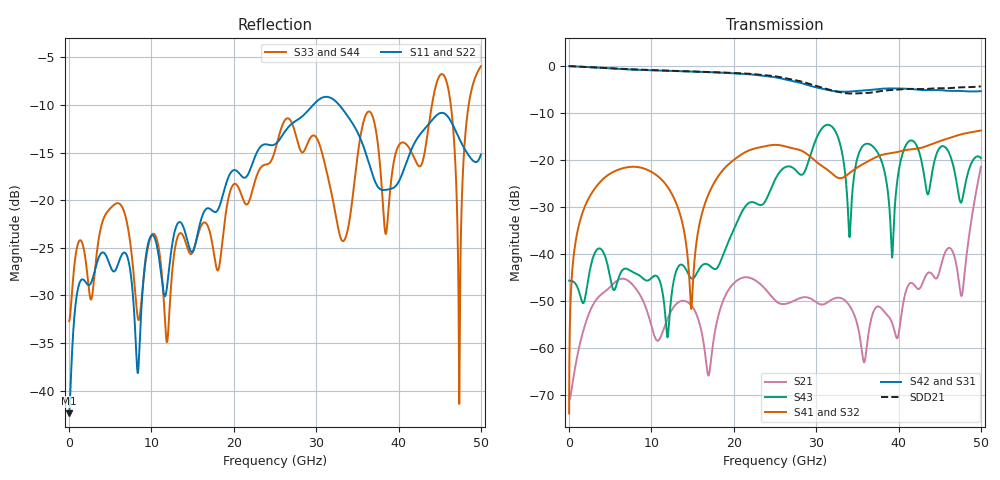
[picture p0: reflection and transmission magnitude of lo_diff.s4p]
!Keysight Technologies,N5245B,MY57181346,A.12.70.07
!Automatic Fixture Removal (AFR)
!Date: Tuesday, November 06, 2018 3:00:35 PM
!S4P File: Measurements: <S11,S12,S13,S14>,
!<S21,S22,S23,S24>,
!<S31,S32,S33,S34>,
!<S41,S42,S43,S44>:
# MHz S  RI  R 50
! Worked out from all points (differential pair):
!   5000 points, 10 MHz to 50 GHz, reference 50 ohm
!   strongest paths, dB at 10 MHz, 12.51 GHz, 25.01 GHz, 37.51 GHz, 50 GHz:
!     S42: 0.0, -1.0, -2.4, -4.9, -5.3
!     S31: 0.0, -1.0, -2.4, -4.9, -5.3
!     S41: -73.9, -27.3, -16.8, -19.2, -13.7
!     S32: -73.9, -27.3, -16.8, -19.2, -13.7
!     S43: -45.7, -47.9, -24.2, -18.5, -19.6
!     S21: -71.0, -51.8, -49.9, -51.2, -21.4
!   taken as a pair (ports 2,1 in; 4,3 out), SDD21 dB: 0.0, -1.0, -2.2, -5.4, -4.3
!   lowest |S11| = -42.4 dB at 10 MHz (marker M1), VSWR 1.02, Z = 50.8 + j0.0342 ohm
!   |S11| at or under -10 dB: start of sweep to 29.63 GHz; 32.8 GHz to end of sweep
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10  0.00759 0.000337  0.000282 4.52e-06  0.9997 -0.00825  0.000108 0.000169
    0.000282 4.52e-06  0.00759 0.000337  0.000108 0.000169  0.9997 -0.00825
    0.9997 -0.00825  0.000108 0.000169  0.0232 0.0004  -0.0052 9.39e-05
    0.000108 0.000169  0.9997 -0.00825  -0.0052 9.39e-05  0.0232 0.0004
3760  -0.0388 -0.0341  -0.00316 -0.00174  -0.9593 -0.0549  0.00271 -0.0581
      -0.00316 -0.00174  -0.0388 -0.0341  0.00271 -0.0581  -0.9593 -0.0549
      -0.9593 -0.0549  0.00271 -0.0581  0.0303 -0.0612  0.0112 -0.0022
      0.00271 -0.0581  -0.9593 -0.0549  0.0112 -0.0022  0.0303 -0.0612
7690  -0.0244 -0.024  -0.000351 -0.00472  0.9194 0.0184  -0.00337 0.0848
      -0.000351 -0.00472  -0.0244 -0.024  -0.00337 0.0848  0.9194 0.0184
      0.9194 0.0184  -0.00337 0.0848  0.0476 -0.00475  0.00491 -0.00416
      -0.00337 0.0848  0.9194 0.0184  0.00491 -0.00416  0.0476 -0.00475
11530  0.031 -0.00763  -0.00152 -0.000564  -0.8943 -0.0475  0.00368 -0.0579
       -0.00152 -0.000564  0.031 -0.00763  0.00368 -0.0579  -0.8943 -0.0475
       -0.8943 -0.0475  0.00368 -0.0579  -0.0164 -0.0233  0.00222 -0.00204
       0.00368 -0.0579  -0.8943 -0.0475  0.00222 -0.00204  -0.0164 -0.0233
15400  0.023 0.0559  -0.00205 -0.00115  0.8732 0.0167  -0.00243 -0.0116
       -0.00205 -0.00115  0.023 0.0559  -0.00243 -0.0116  0.8732 0.0167
       0.8732 0.0167  -0.00243 -0.0116  -0.0215 0.0562  0.00562 -0.00207
       -0.00243 -0.0116  0.8732 0.0167  0.00562 -0.00207  -0.0215 0.0562
19150  -0.056 0.1119  -0.000809 0.00376  -0.8444 -0.0637  -0.00603 0.0863
       -0.000809 0.00376  -0.056 0.1119  -0.00603 0.0863  -0.8444 -0.0637
       -0.8444 -0.0637  -0.00603 0.0863  0.0401 0.0829  0.0122 -0.00172
       -0.00603 0.0863  -0.8444 -0.0637  0.0122 -0.00172  0.0401 0.0829
50000  0.1733 -0.0104  0.0819 -0.0214  -0.541 -0.00916  0.0295 0.2042
       0.0819 -0.0214  0.1733 -0.0104  0.0295 0.2042  -0.541 -0.00916
       -0.541 -0.00916  0.0295 0.2042  -0.2713 -0.4263  0.0255 -0.1015
       0.0295 0.2042  -0.541 -0.00916  0.0255 -0.1015  -0.2713 -0.4263
